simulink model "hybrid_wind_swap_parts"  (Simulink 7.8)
settings: Solver=ode3  SolverMode=SingleTasking  StartTime=0.0  StopTime=inf  FixedStep=Ts  RelTol=1e-3
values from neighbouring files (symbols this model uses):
  Ampl_chirp = maxoutputvoltage/4    (= 1.25)    [measurements.m]
  Ampl_chirp_U = maxoutputvoltage *amp_gain_factor*Bl/Re/(2*pi*fstop)*Sd/Mms    [measurements.m]
  gamma_cte = 0.7    [single_reed.m]
  micpreampsensitivity = -0.0025726    [hybrid_wind.m]    (also in measurements.m)
  sweep_time = runtime    (= 20)    [measurements.m]
  Ts = 25e-6    (= 2.5e-05)    [hybrid_wind.m]    (also in measurements.m)
  wr = 2*pi*140*0.7    (= 615.752160104)    [lip_reed.m]    (also in single_reed.m = 15707.9632679)
  Zc = rho*c/St    (= 2615281.00417)    [hybrid_wind.m]
undefined symbols (not defined in the file or in its folder): bal2gamm, Bl, cell2mat, He_d, HLSinv_PD_den, HLSinv_PD_num, HRreed_G, HRreed_G_zm1, lsr2zeta, Re, Sd, sigbuilder_block, wLP, zetaLP, zetar
libraries: instrumentlib x3, dspsrcs4 x2, simulink x2, dspmlti4 x1

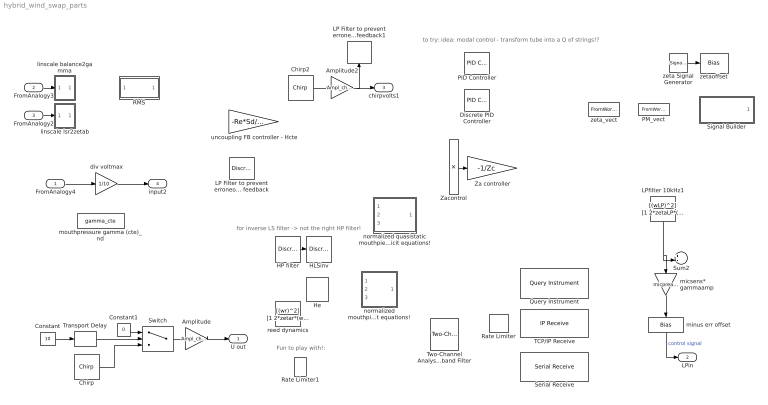
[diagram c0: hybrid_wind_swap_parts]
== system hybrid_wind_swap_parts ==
  note: to try: idea: modal control - transform tube into a Q of strings!?
  note: for inverse LS filter -> not the right HP filter!
  note: Fun to play with!:
  FromAnalogy4 : Inport
  FromAnalogy3 : Inport  Port=2  SampleTime=Ts*1000
  FromAnalogy2 : Inport  Port=3  SampleTime=Ts*500
  Amplitude : Gain  Gain=Ampl_chirp
  Amplitude2 : Gain  Gain=Ampl_chirp_U
  Chirp : dspsrcs4/Chirp  sweep=Linear  mode=Unidirectional  f0=fstart  f1=fstop  t1=sweep_time  Tsweep=sweep_time  phase=pi/2  Ts=Ts  spf=1  datatype=Single
  Chirp2 : dspsrcs4/Chirp  sweep=Linear  mode=Unidirectional  f0=fstart  f1=fstop  t1=sweep_time  Tsweep=sweep_time  phase=pi/2  Ts=Ts  spf=1  datatype=Double
  Constant : Constant  Value=10
  Constant1 : Constant  Value=0
  Discrete PID Controller : simulink/Continuous/PID Controller  Controller=PID  TimeDomain=Discrete-time  SampleTime=1  IntegratorMethod=Forward Euler  FilterMethod=Forward Euler  Form=Parallel  P=1  I=1  D=0  N=100  InitialConditionSource=internal  InitialConditionForIntegrator=0  InitialConditionForFilter=0  ExternalReset=none  LimitOutput=off  UpperSaturationLimit=inf  LowerSaturationLimit=-inf  LinearizeAsGain=off  AntiWindupMode=none  Kb=1  TrackingMode=off  Kt=1  PParamMin=[]  PParamMax=[]  IParamMin=[]  IParamMax=[]  DParamMin=[]  DParamMax=[]  NParamMin=[]  NParamMax=[]  KbParamMin=[]  KbParamMax=[]  KtParamMin=[]  KtParamMax=[]  POutMin=[]  POutMax=[]  IOutMin=[]  IOutMax=[]  DOutMin=[]  DOutMax=[]  NOutMin=[]  NOutMax=[]  KbOutMin=[]  KbOutMax=[]  KtOutMin=[]  KtOutMax=[]  IntegratorOutMin=[]  IntegratorOutMax=[]  FilterOutMin=[]  FilterOutMax=[]  SumOutMin=[]  SumOutMax=[]  SumI1OutMin=[]  SumI1OutMax=[]  SumI2OutMin=[]  SumI2OutMax=[]  SumI3OutMin=[]  SumI3OutMax=[]  SumDOutMin=[]  SumDOutMax=[]  SaturationOutMin=[]  SaturationOutMax=[]  IntegratorContinuousStateAttributes=''  IntegratorStateMustResolveToSignalObject=off  IntegratorRTWStateStorageClass=Auto  FilterContinuousStateAttributes=''  FilterStateMustResolveToSignalObject=off  FilterRTWStateStorageClass=Auto
  HLSinv : DiscreteTransferFcn  Numerator=HLSinv_PD_num{1}  Denominator=HLSinv_PD_den{1}  SampleTime=Ts
  HP filter : DiscreteTransferFcn  Numerator=HdHP.ScaleValues(1)*HdHP.sosMatrix(1:end/2)  Denominator=HdHP.ScaleValues(2)*HdHP.sosMatrix(1+end/2:end)  SampleTime=Ts
  He : DiscreteTransferFcn  Numerator=cell2mat(He_d.num)  Denominator=cell2mat(He_d.den)  SampleTime=Ts
  LP Filter to prevent erroneous high freq feedback : DiscreteFilter  Numerator=HdLP.ScaleValues(1)*HdLP.sosMatrix(1:end/2)  Denominator=HdLP.ScaleValues(2)*HdLP.sosMatrix(1+end/2:end)  SampleTime=Ts
  LP Filter to prevent erroneous high freq feedback1 : DiscreteFilter  Numerator=HdLP.ScaleValues(1)*HdLP.sosMatrix(1:end/2)  Denominator=HdLP.ScaleValues(2)*HdLP.sosMatrix(1+end/2:end)  SampleTime=Ts
  LPfilter 10kHz1 : TransferFcn  Numerator=[(wLP)^2]  Denominator=[1 2*zetaLP*(wLP) (wLP)^2]
  PID Controller : simulink/Continuous/PID Controller  Controller=PID  TimeDomain=Continuous-time  SampleTime=1  IntegratorMethod=Forward Euler  FilterMethod=Forward Euler  Form=Parallel  P=1  I=1  D=0  N=100  InitialConditionSource=internal  InitialConditionForIntegrator=0  InitialConditionForFilter=0  ExternalReset=none  LimitOutput=off  UpperSaturationLimit=inf  LowerSaturationLimit=-inf  LinearizeAsGain=off  AntiWindupMode=none  Kb=1  TrackingMode=off  Kt=1  PParamMin=[]  PParamMax=[]  IParamMin=[]  IParamMax=[]  DParamMin=[]  DParamMax=[]  NParamMin=[]  NParamMax=[]  KbParamMin=[]  KbParamMax=[]  KtParamMin=[]  KtParamMax=[]  POutMin=[]  POutMax=[]  IOutMin=[]  IOutMax=[]  DOutMin=[]  DOutMax=[]  NOutMin=[]  NOutMax=[]  KbOutMin=[]  KbOutMax=[]  KtOutMin=[]  KtOutMax=[]  IntegratorOutMin=[]  IntegratorOutMax=[]  FilterOutMin=[]  FilterOutMax=[]  SumOutMin=[]  SumOutMax=[]  SumI1OutMin=[]  SumI1OutMax=[]  SumI2OutMin=[]  SumI2OutMax=[]  SumI3OutMin=[]  SumI3OutMax=[]  SumDOutMin=[]  SumDOutMax=[]  SaturationOutMin=[]  SaturationOutMax=[]  IntegratorContinuousStateAttributes=''  IntegratorStateMustResolveToSignalObject=off  IntegratorRTWStateStorageClass=Auto  FilterContinuousStateAttributes=''  FilterStateMustResolveToSignalObject=off  FilterRTWStateStorageClass=Auto
  PM_vect : FromWorkspace  VariableName=PM_vect  SampleTime=0
  Query Instrument : instrumentlib/Query Instrument  sampleTime=1  isWorkspaceObject=off  timeout=10  inputBufferSize=512  protocol=Serial  serialPort=COM1  baudRate=9600  gpibVendor=Advantech  boardIndex=0  primaryAddress=1  secondaryAddress=0  visaVendor=Agilent  visaSerialPort=0  chassisIndex=0  logicalAddress=0  tcpRemoteHost='127.0.0.1'  tcpRemotePort=4500  udpRemoteHost='127.0.0.1'  udpRemotePort=9090  visaTCPBoardIndex=0  visaTCPRemoteHost='127.0.0.1'  usbBoardIndex=0  usbManufID=0  usbModelCode=0  usbSerialNumber=0  initAction=None  initCommand='DATA:SOURCE CH1'  initFunction=get  queryCommand='curve?'  responseFormat=ASCII  asciiFormatting='%d,'  precision=8-bit integer  byteOrder=Little endian  valuesToRead=1  removeBytes=off  afterOutputAction=Repeat query for new data  enableFrames=off  frameSize=1
  RMS : Subsystem
  Rate Limiter : RateLimiter  SampleTimeMode=inherited
  Rate Limiter1 : RateLimiter  RisingSlewLimit=350  FallingSlewLimit=-350  SampleTimeMode=inherited
  Serial Receive : instrumentlib/Serial Receive  ComPortMenu=<Please select a port...>  ComPort=<Please select a port...>  Terminator=<none>  DataSize=[1 1]  DataType=uint8  EnableBlockingMode=on  ActionDataUnavailable=Output last received value  CustomValue=0  SampleTime=0.01
  Signal Builder : Subsystem  Tag=STV Subsys  LoadFcn=sigbuilder_block('load');  StartFcn=sigbuilder_block('start');  StopFcn=sigbuilder_block('stop');  ClipboardFcn=sigbuilder_block('clipboard');
  Sum2 : Sum  Inputs=+-|
  Switch : Switch  Threshold=1
  TCP/IP Receive : instrumentlib/TCP//IP Receive  Port=80  DataSize=[1 1]  EnableBlockingMode=on  Timeout=10  SampleTime=0.01  DataType=uint8  ByteOrder=BigEndian
  Transport Delay : TransportDelay  DelayTime=sweep_time  BufferSize=8
  Two-Channel Analysis Subband Filter : dspmlti4/Two-Channel Analysis Subband Filter  lpf="[0.0352   -0.0854   -0.1350   0.4599   0.8069   0.3327]"  hpf="[-0.3327    0.8069   -0.4599   -0.1350    0.0854    0.0352]"  framing=Enforce single-rate processing  InputProcessing=Columns as channels (frame based)  firstCoeffDataTypeStr=Inherit: Same word length as input  firstCoeffLastDataTypeStr=Inherit: Same word length as input  firstCoeffMin=[]  firstCoeffMax=[]  outputDataTypeStr=Inherit: Same as accumulator  outputLastDataTypeStr=Inherit: Same as accumulator  outputMin=[]  outputMax=[]  roundingMode=Floor  overflowMode=off
  Za controller : Gain  Gain=-1/Zc
  Zacontrol : Product  Inputs=**
  div voltmax : Gain  Gain=1/10
  linscale balance2gamma : Subsystem
  linscale lsr2zetab : Subsystem
  micsens* gammaamp : Gain  Gain=micpreampsensitivity/5
  minus err offset : Bias  Bias=-0.1
  mouthpressure gamma (cte)_nd : Constant  Value=gamma_cte
  normalized mouthpiece model -not optimized for implicit equations! : Subsystem
  normalized quasistatic mouthpiece model - optimized for implicit equations! : Subsystem
  reed dynamics : TransferFcn  Numerator=[(wr)^2]  Denominator=[1 2*zetar*(wr) (wr)^2]
  uncoupling FB controller - Hcte : Gain  Gain=-Re*Sd/Bl
  zeta Signal Generator : SignalGenerator  WaveForm=sawtooth  Amplitude=(0.6-0.1)/2  Frequency=0.2
  zeta_vect : FromWorkspace  VariableName=zeta_vect  SampleTime=0
  zetaoffset : Bias  Bias=0.1+(0.6-0.1)/2
  U out : Outport
  LPin : Outport  Port=2
  chirpvolts1 : Outport  Port=3
  input2 : Outport  Port=4
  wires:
  Constant/1 -> Transport Delay/1
  Transport Delay/1 -> Switch/2
  Constant1/1 -> Switch/1
  Switch/1 -> Amplitude/1
  Chirp/1 -> Switch/3
  Amplitude/1 -> U out/1
  ? -> LPfilter 10kHz1/1, Sum2/1
  ? -> ?
  LPfilter 10kHz1/1 -> Sum2/2, micsens* gammaamp/1
  micsens* gammaamp/1 -> minus err offset/1
  minus err offset/1 -> LPin/1  "control signal"
  zeta Signal Generator/1 -> zetaoffset/1
  Zacontrol/1 -> Za controller/1
  Chirp2/1 -> Amplitude2/1
  Amplitude2/1 -> chirpvolts1/1, LP Filter to prevent erroneous high freq feedback1/1
  HP filter/1 -> HLSinv/1
  FromAnalogy4/1 -> div voltmax/1
  div voltmax/1 -> input2/1
  FromAnalogy3/1 -> linscale balance2gamma/1(In1)
  FromAnalogy2/1 -> linscale lsr2zetab/1(In1)

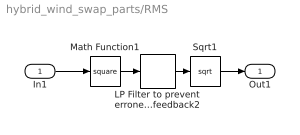
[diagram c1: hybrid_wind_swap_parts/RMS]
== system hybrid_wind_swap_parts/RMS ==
  In1 : Inport
  LP Filter to prevent erroneous high freq feedback2 : DiscreteFilter  Numerator=HdLPRMS.ScaleValues(1)*HdLPRMS.sosMatrix(1:end/2)  Denominator=HdLPRMS.ScaleValues(2)*HdLPRMS.sosMatrix(1+end/2:end)  SampleTime=Ts
  Math Function1 : Math  Operator=square
  Sqrt1 : Sqrt
  Out1 : Outport
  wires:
  Math Function1/1 -> LP Filter to prevent erroneous high freq feedback2/1
  LP Filter to prevent erroneous high freq feedback2/1 -> Sqrt1/1
  In1/1 -> Math Function1/1
  Sqrt1/1 -> Out1/1

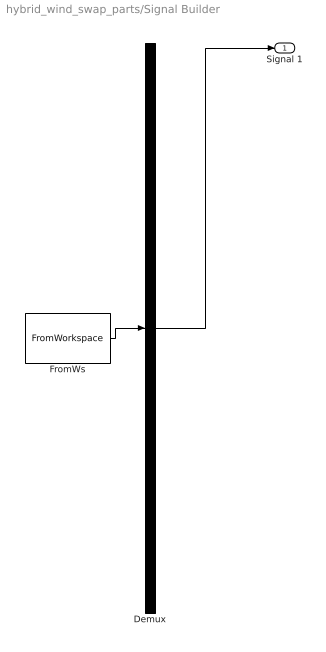
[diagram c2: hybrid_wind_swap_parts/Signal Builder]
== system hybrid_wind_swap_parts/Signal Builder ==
  Demux : Demux  Tag=STV Demux  Outputs=1
  FromWs : FromWorkspace  Tag=STV FromWs  VariableName=tuvar  SampleTime=0  SigBuilderData=DataTag0  VnvData=DataTag1
  Signal 1 : Outport  Tag=STV Outport
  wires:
  Demux/1 -> Signal 1/1
  FromWs/1 -> Demux/1

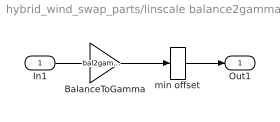
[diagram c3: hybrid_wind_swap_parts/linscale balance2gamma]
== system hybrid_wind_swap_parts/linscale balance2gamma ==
  In1 : Inport
  BalanceToGamma : Gain  Gain=bal2gamm.slope
  min offset : Bias  Bias=bal2gamm.offset
  Out1 : Outport
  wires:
  BalanceToGamma/1 -> min offset/1
  min offset/1 -> Out1/1
  In1/1 -> BalanceToGamma/1

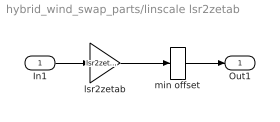
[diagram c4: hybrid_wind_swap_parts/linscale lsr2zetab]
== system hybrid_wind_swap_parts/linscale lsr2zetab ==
  In1 : Inport
  lsr2zetab : Gain  Gain=lsr2zeta.slope
  min offset : Bias  Bias=lsr2zeta.offset
  Out1 : Outport
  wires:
  lsr2zetab/1 -> min offset/1
  min offset/1 -> Out1/1
  In1/1 -> lsr2zetab/1

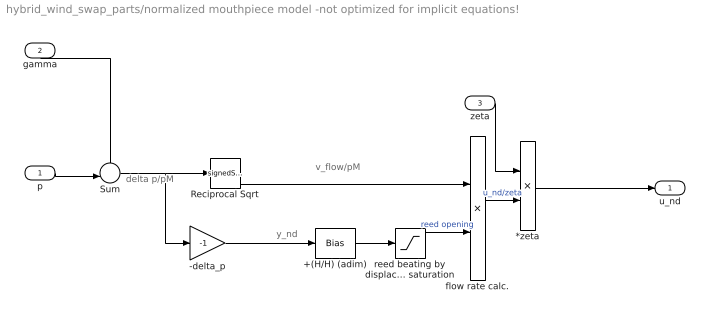
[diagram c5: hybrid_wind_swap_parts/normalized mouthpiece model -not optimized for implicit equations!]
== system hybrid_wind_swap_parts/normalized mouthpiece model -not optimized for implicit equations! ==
  note: v_flow/pM
  note: y_nd
  note: delta p/pM
  p : Inport
  gamma : Inport  Port=2
  zeta : Inport  Port=3
  *zeta : Product  Inputs=**
  +(H/H) (adim) : Bias  Bias=1
  -delta_p : Gain  Gain=-1
  Reciprocal Sqrt : Sqrt  Operator=signedSqrt
  Sum : Sum  Inputs=+-|
  flow rate calc. : Product
  reed beating by displacement saturation : Saturate  UpperLimit=100  LowerLimit=0
  u_nd : Outport
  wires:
  gamma/1 -> Sum/1
  p/1 -> Sum/2
  zeta/1 -> *zeta/1
  +(H/H) (adim)/1 -> reed beating by displacement saturation/1
  reed beating by displacement saturation/1 -> flow rate calc./2  "reed opening"
  Reciprocal Sqrt/1 -> flow rate calc./1
  flow rate calc./1 -> *zeta/2  "u_nd/zeta"
  *zeta/1 -> u_nd/1
  Sum/1 -> Reciprocal Sqrt/1, -delta_p/1
  -delta_p/1 -> +(H/H) (adim)/1

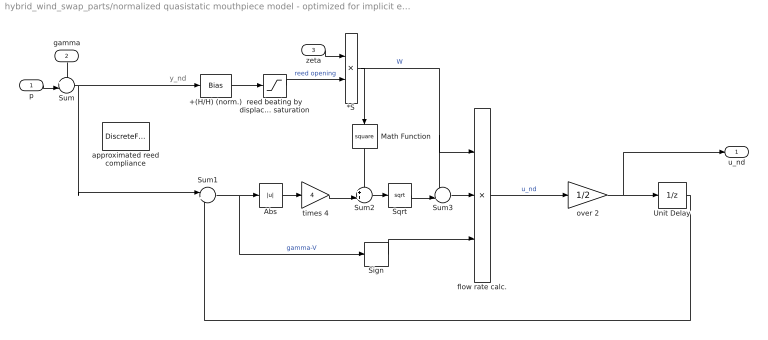
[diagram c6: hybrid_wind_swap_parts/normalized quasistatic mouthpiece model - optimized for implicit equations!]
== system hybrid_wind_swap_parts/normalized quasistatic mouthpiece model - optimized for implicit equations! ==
  note: y_nd
  p : Inport
  gamma : Inport  Port=2
  zeta : Inport  Port=3
  *S : Product  Inputs=**
  +(H/H) (norm.) : Bias  Bias=1
  Abs : Abs
  Math Function : Math  Operator=square
  Sign : Signum
  Sqrt : Sqrt
  Sum : Sum  Inputs=+-|
  Sum1 : Sum  Inputs=|++
  Sum2 : Sum  Inputs=++|
  Sum3 : Sum  Inputs=-+|
  Unit Delay : UnitDelay  SampleTime=-1
  approximated reed compliance : DiscreteFilter  Numerator=HRreed_G_zm1.num  Denominator=HRreed_G.den  SampleTime=Ts  a0EqualsOne=on
  flow rate calc. : Product  Inputs=3
  over 2 : Gain  Gain=1/2
  reed beating by displacement saturation : Saturate  UpperLimit=100  LowerLimit=0
  times 4 : Gain  Gain=4
  u_nd : Outport
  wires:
  gamma/1 -> Sum/1
  p/1 -> Sum/2
  zeta/1 -> *S/1
  +(H/H) (norm.)/1 -> reed beating by displacement saturation/1
  Sum2/1 -> Sqrt/1
  Sum1/1 -> Abs/1, Sign/1  "gamma-V"
  reed beating by displacement saturation/1 -> *S/2  "reed opening"
  Sum/1 -> Sum1/1, +(H/H) (norm.)/1
  *S/1 -> flow rate calc./1, Sum3/1, Math Function/1  "W"
  flow rate calc./1 -> over 2/1  "u_nd"
  Sqrt/1 -> Sum3/2
  Sum3/1 -> flow rate calc./2
  over 2/1 -> u_nd/1, Unit Delay/1
  Math Function/1 -> Sum2/1
  Abs/1 -> times 4/1
  times 4/1 -> Sum2/2
  Sign/1 -> flow rate calc./3
  Unit Delay/1 -> Sum1/2
